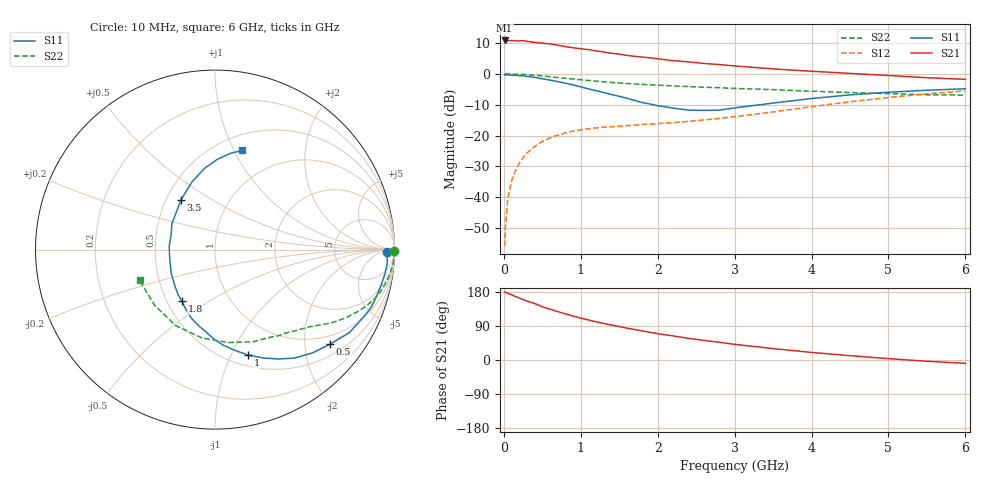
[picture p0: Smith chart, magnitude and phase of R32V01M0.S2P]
! SIEMENS Small Signal Semiconductors
! BFR181
! Si NPN RF Bipolar Junction Transistor in SOT23
! VCE = 2 V  IC = 1 mA
! Common Emitter S-Parameters:  May  1996
# GHz  S  MA  R  50
!  f  S11  S21  S12  S22
! GHz  MAG  ANG  MAG  ANG  MAG  ANG  MAG  ANG
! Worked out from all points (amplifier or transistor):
!   36 points, 10 MHz to 6 GHz, reference 50 ohm
!   highest |S21| = 10.8 dB at 10 MHz (marker M1)
!   |S21| within 3 dB of that: start of sweep to 1.103 GHz
!   unconditionally stable (mu >= 1): 1.992 GHz to 3.687 GHz
!   at 250 MHz: K = 0.16, MSG = 19.0 dB, |S12| = -27.2 dB
!   at 1.4 GHz: K = 0.78, MSG = 11.9 dB, |S12| = -17.1 dB
!   at 6 GHz: K = 0.88, MSG = 1.9 dB, |S12| = -5.5 dB
!   lowest NFmin = 1.30 dB at 450 MHz
!   S11 on the Smith chart (normalised r, x): 10 MHz: 42, -14; 500 MHz: 0.77, -2.59; 1 GHz: 0.61, -1.16; 1.8 GHz: 0.59, -0.39; 3.5 GHz: 0.60, +0.37; 6 GHz: 0.66, +1.08
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0.01  0.9584 -0.8  3.486 179.5  0.0016 95.3  0.998 -0.5
0.02  0.9579 -1.7  3.44 178.3  0.0032 90.9  0.9974 -0.8
0.05  0.9635 -4.1  3.447 176.1  0.0092 86.9  0.9972 -2.0
0.1  0.9568 -8.1  3.483 172.4  0.0182 84.8  0.9966 -3.7
0.15  0.9463 -12.0  3.43 167.5  0.0267 81.0  0.99 -5.8
0.25  0.9276 -20.3  3.457 159.6  0.0438 76.6  0.9777 -9.5
0.5  0.8298 -39.4  3.152 140.6  0.0799 65.4  0.9258 -17.6
0.6  0.7915 -46.6  3.064 134.1  0.0914 61.5  0.899 -20.5
0.7  0.7503 -53.6  2.924 127.8  0.1011 57.9  0.872 -23.1
0.9  0.6631 -65.7  2.649 115.9  0.1181 52.3  0.8257 -27.2
1  0.6157 -72.6  2.563 110.6  0.1233 49.9  0.8033 -29.0
1.1  0.5703 -79.1  2.471 105.7  0.1288 48.2  0.782 -30.8
1.4  0.4611 -96.3  2.161 92.1  0.1389 44.3  0.7268 -35.2
1.6  0.4027 -109.4  1.991 84.0  0.1447 43.2  0.6986 -37.5
1.8  0.342 -122.7  1.874 76.8  0.151 43.1  0.6759 -39.8
2.2  0.2789 -150.6  1.637 63.5  0.1618 44.7  0.6388 -44.9
2.4  0.2578 -168.2  1.567 57.2  0.1693 46.2  0.622 -47.4
2.8  0.2582 161.1  1.417 46.7  0.1893 48.6  0.5961 -53.6
3.5  0.3359 124.2  1.205 30.1  0.2411 50.8  0.5548 -67.8
4.5  0.4566 97.3  1.019 11.4  0.352 46.3  0.4976 -98.5
5.5  0.543 81.0  0.867 -3.3  0.4744 33.7  0.4577 -137.5
6  0.5733 74.5  0.815 -8.8  0.5285 25.9  0.4533 -157.9
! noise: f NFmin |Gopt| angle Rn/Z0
0.45  1.3  0.7  18  0.5
0.9  1.4  0.6  39  0.52
1.8  1.85  0.4  81  0.47
